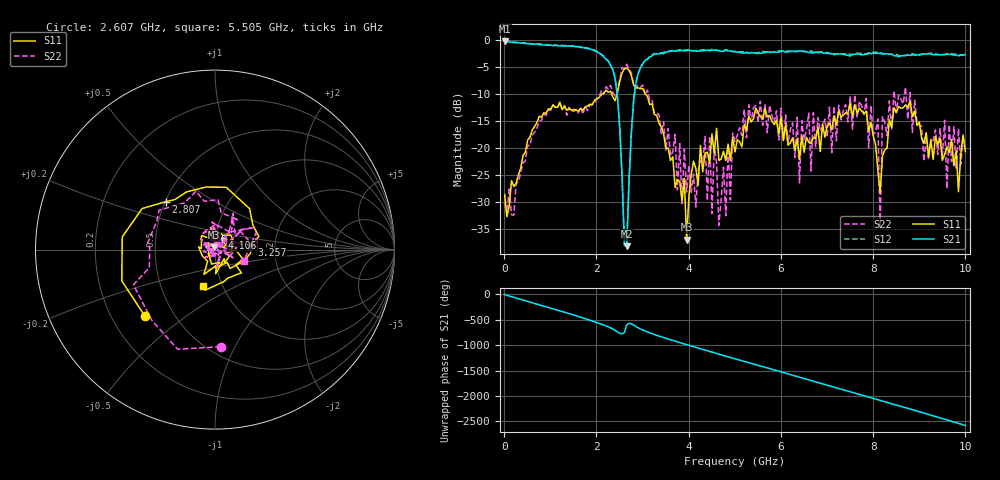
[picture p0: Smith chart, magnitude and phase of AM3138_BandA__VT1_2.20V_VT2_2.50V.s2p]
! Date/Time: Tue, Nov 13, 2018 4:42 PM
! Network Analyzer: Agilent Technologies E8364B Rev: A.07.50.67
! Sweep from 0.010 to 10.000 GHz, 201 Points, Sweep Type: LIN
! Power Supply: 2.201 V, 0.000 A
# Hz S DB R 50
!freq MagS11 AngS11 MagS21 AngS21 MagS12 AngS12 MagS22 AngS22
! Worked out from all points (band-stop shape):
!   201 points, 10 MHz to 10 GHz, reference 50 ohm
!   highest |S21| = -0.32 dB at 10 MHz (marker M1); lowest = -38.2 dB at 2.657 GHz (marker M2)
!   |S21| within 3 dB of the highest: start of sweep to 2.175 GHz; 3.147 GHz to end of sweep
!   lowest |S11| = -37.0 dB at 3.956 GHz (marker M3), VSWR 1.03, Z = 49.4 + j1.29 ohm
!   |S11| at or under -10 dB: start of sweep to 2.136 GHz; 2.329 GHz to 2.449 GHz (120.5 MHz wide, 5.04 % of centre); 3.056 GHz to end of sweep
!   |S22| runs from -34.9 to -4.5 dB; largest |S21 - S12| = 0.031
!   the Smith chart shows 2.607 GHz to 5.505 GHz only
!   S11 on the Smith chart (normalised r, x): 2.607 GHz: 0.34, -0.36; 2.807 GHz: 0.50, +0.32; 3.257 GHz: 1.50, +0.08; 4.106 GHz: 1.07, +0.14; 5.505 GHz: 0.81, -0.34
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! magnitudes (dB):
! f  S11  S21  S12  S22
! 10 MHz  -28.6  -0.3  -0.1  -30.1
! 1.708 GHz  -13.1  -1.4  -1.4  -13.8
! 2.408 GHz  -11.3  -7.3  -7.2  -10.4
! 2.607 GHz  -5.4  -38.1  -37.8  -5.3
! 2.657 GHz  -5.2  -38.2  -38.2  -4.5
! 2.807 GHz  -8.4  -11.3  -11.1  -8.4
! 3.257 GHz  -13.8  -2.7  -2.6  -13.6
! 3.357 GHz  -15.5  -2.6  -2.5  -13.8
! 3.956 GHz  -37.0  -2.0  -1.9  -28.2
! 4.106 GHz  -22.5  -2.0  -2.1  -24.8
! 4.456 GHz  -22.8  -2.0  -2.0  -17.9
! 4.655 GHz  -22.3  -2.0  -2.0  -34.3
! 5.005 GHz  -20.8  -2.2  -2.2  -18.8
! 5.505 GHz  -13.5  -2.5  -2.3  -15.3
! 6.404 GHz  -22.2  -2.1  -2.0  -26.5
! 6.703 GHz  -18.0  -2.5  -2.3  -13.5
! 7.952 GHz  -15.3  -2.6  -2.4  -12.2
! 8.102 GHz  -24.1  -2.5  -2.3  -14.7
! 8.152 GHz  -28.3  -2.5  -2.4  -34.9
! 8.202 GHz  -21.5  -2.7  -2.5  -14.2
! 8.352 GHz  -14.8  -2.7  -2.7  -11.3
! 10 GHz  -20.7  -2.8  -2.7  -19.0
